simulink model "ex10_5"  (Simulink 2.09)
settings: Solver=VariableStepDiscrete  StartTime=0.0  StopTime=3  RelTol=1e-3  AbsTol=1e-6

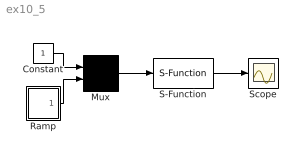
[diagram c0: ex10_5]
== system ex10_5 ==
  Constant : Constant  Value=1
  Mux : Mux  Inputs=2
  Ramp : Subsystem  mask( Ramp){}
      mask help: ramp
      mask init:
      | slope=@1;start=@2;X0=@3;
  S-Function : S-Function  FunctionName=s_xmp1
  Scope : Scope
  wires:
  S-Function/1 -> Scope/1
  Mux/1 -> S-Function/1
  Ramp/1(out1) -> Mux/2
  Constant/1 -> Mux/1

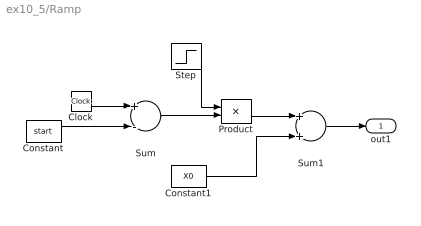
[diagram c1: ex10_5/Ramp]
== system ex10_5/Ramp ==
  Clock : Clock
  Constant : Constant  Value=start
  Constant1 : Constant  Value=X0
  Product : Product  Inputs=2
  Step : Step  Time=start  Before=0  After=slope
  Sum : Sum  Inputs=+-
  Sum1 : Sum  Inputs=++
  out1 : Outport  Port=1  InitialOutput=0
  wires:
  Sum1/1 -> out1/1
  Constant1/1 -> Sum1/2
  Product/1 -> Sum1/1
  Step/1 -> Product/1
  Clock/1 -> Sum/1
  Constant/1 -> Sum/2
  Sum/1 -> Product/2
